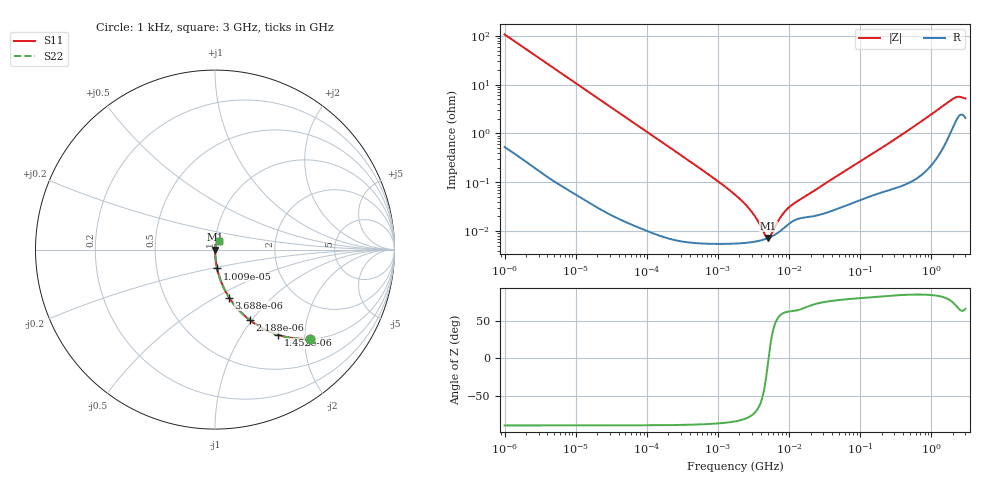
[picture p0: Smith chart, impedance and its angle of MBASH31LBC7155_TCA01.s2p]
! MBASH31LBC7155_TCA01  S-PARAMETER MODEL  ( Standard Model )
! Model Generated by TAIYO YUDEN Corporation (http://www.ty-top.com)
! Version 1.0
! TAIYO YUDEN Control No. 220601
! Copyright(c) 2019 TAIYO YUDEN CO.,LTD. All Rights Reserved.
! Product Description (link to TY-COMPAS)
! https://ds.yuden.co.jp/TYCOMPAS/or/detail?pn=MBASH31LBC7155KTCA01&u=M
! Products Name : Multilayer Ceramic Capacitors
! Characteristics :
!  Capacitance : 1.5 [uF] , Rated Voltage : 100 [V] , TCC : X7S
!  Case Size : 3.2 x 1.6 / 0.126 x 0.063 [mm/inch] , Thickness : 1.6 / 0.063 [mm/inch]
!  (Conditions: Temperature = 25 [degC] , DC Bias Voltage = 0 [V])
! External Node Assignments :
!  1  o---| |---o  2
! GND o---------o GND
! Frequency Range : 1kHz  -  3GHz  [ 401 STEP ]
# MHZ S RI R 50
! Freq[MHz].  S11 Real  S11 Imag  S21 Real  S21 Imag  S12 Real  S12 Imag  S22 Real  S22 Imag
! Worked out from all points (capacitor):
!   401 points, 1 kHz to 3 GHz, reference 50 ohm
!   read as one part in series: C = 1.49 uF near 1.077 kHz
!   lowest |Z| = 7.24 mohm at 5.107 MHz (marker M1)
!   series resonance near 5.129 MHz, so ESL is about 650 pH
!   S11 on the Smith chart (normalised r, x): 1 kHz: 1.01, -2.13; 1.452 kHz: 1.01, -1.47; 2.188 kHz: 1.00, -0.98; 3.688 kHz: 1.00, -0.58; 10.09 kHz: 1.00, -0.21; 3 GHz: 1.04, +0.10
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0.001  0.5314 -0.4965  0.4686 0.4965  0.4686 0.4965  0.5314 -0.4965
0.001452  0.3513 -0.4749  0.6487 0.4749  0.6487 0.4749  0.3513 -0.4749
0.002188  0.1936 -0.3927  0.8064 0.3927  0.8064 0.3927  0.1936 -0.3927
0.003688  0.0787 -0.2669  0.9213 0.2669  0.9213 0.2669  0.0787 -0.2669
0.010091  0.0117 -0.105  0.9883 0.105  0.9883 0.105  0.0117 -0.105
0.01216  0.00819 -0.0875  0.9918 0.0875  0.9918 0.0875  0.00819 -0.0875
0.033275  0.00125 -0.0323  0.9988 0.0323  0.9988 0.0323  0.00125 -0.0323
0.147855  0.000135 -0.00731  0.9999 0.00731  0.9999 0.00731  0.000135 -0.00731
0.791611  5.66e-05 -0.00134  0.9999 0.00134  0.9999 0.00134  5.66e-05 -0.00134
1.732051  5.58e-05 -0.000555  0.9999 0.000555  0.9999 0.000555  5.58e-05 -0.000555
2.919173  5.92e-05 -0.000251  0.9999 0.000251  0.9999 0.000251  5.92e-05 -0.000251
4.238263  6.6e-05 -8.1e-05  0.9999 8.1e-05  0.9999 8.1e-05  6.6e-05 -8.1e-05
4.566395  6.82e-05 -4.91e-05  0.9999 4.91e-05  0.9999 4.91e-05  6.82e-05 -4.91e-05
5.106836  7.24e-05 -1.79e-06  0.9999 1.79e-06  0.9999 1.79e-06  7.24e-05 -1.79e-06
5.928204  8.02e-05 6.1e-05  0.9999 -6.1e-05  0.9999 -6.1e-05  8.02e-05 6.1e-05
7.988506  0.000108 0.000187  0.9999 -0.000187  0.9999 -0.000187  0.000108 0.000187
9.991309  0.000142 0.000275  0.9999 -0.000275  0.9999 -0.000275  0.000142 0.000275
21.06097  0.0002 0.000598  0.9998 -0.000598  0.9998 -0.000598  0.0002 0.000598
256.0921  0.000732 0.00636  0.9993 -0.00636  0.9993 -0.00636  0.000732 0.00636
1990.675  0.0152 0.0479  0.9848 -0.0479  0.9848 -0.0479  0.0152 0.0479
2398.636  0.0242 0.0496  0.9758 -0.0496  0.9758 -0.0496  0.0242 0.0496
3000  0.0225 0.0457  0.9775 -0.0457  0.9775 -0.0457  0.0225 0.0457
